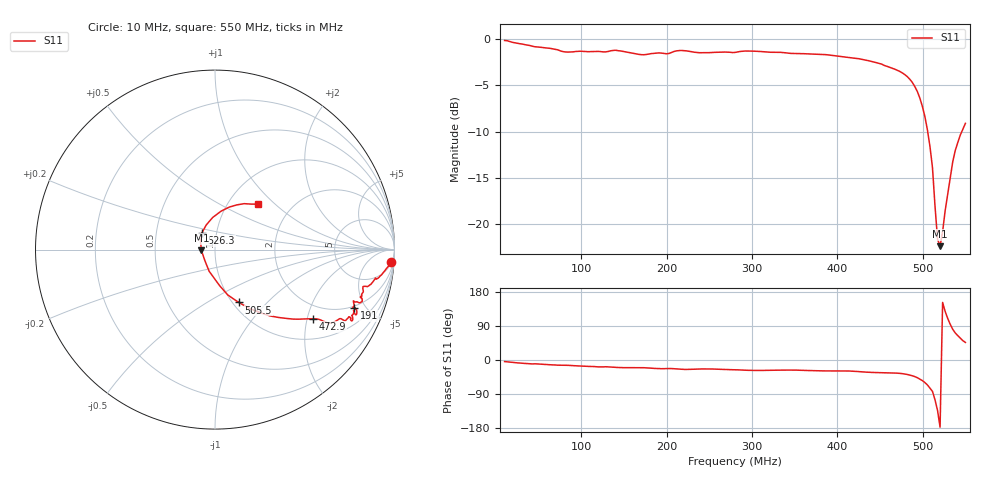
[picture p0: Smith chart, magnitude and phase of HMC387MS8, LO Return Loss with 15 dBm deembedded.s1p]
!Hittite Microwave Corporation
!12 Elizabeth Drive
!Chelmsford, MA 01824
!Tel: 978-250-3343
!Fax: 978-250-3373
!Device: HMC387MS8, 450-500 MHz, GaAs MMIC High IP3 Mixer in 8-lead plastic SMT package
!Misc: LO Return Loss with 15 dBm, Room
# MHZ S MA R 50
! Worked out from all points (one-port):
!   183 points, 10 MHz to 550 MHz, reference 50 ohm
!   lowest |S11| = -22.4 dB at 520.3 MHz (marker M1), VSWR 1.16, Z = 42.9 - j0.309 ohm
!   |S11| at or under -10 dB: 505.8 MHz to 545.8 MHz (40 MHz wide, 7.61 % of centre)
!   S11 on the Smith chart (normalised r, x): 10 MHz: 7, -26; 191 MHz: 1.87, -4.16; 472.9 MHz: 1.56, -2.18; 505.5 MHz: 1.07, -0.70; 526.3 MHz: 0.85, +0.16; 550 MHz: 1.37, +0.79
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10  0.982 -4.1
36.703  0.927 -9.6
78.242  0.855 -13.8
146.484  0.861 -20.1
173.187  0.822 -20.4
190.989  0.841 -22.8
202.857  0.836 -22.5
214.725  0.866 -24.2
250.33  0.844 -23.6
280  0.846 -25.7
303.736  0.859 -27.5
348.242  0.835 -26.6
380.879  0.827 -28.7
416.484  0.791 -29.3
440.22  0.756 -32.8
472.857  0.669 -35.2
484.725  0.607 -39.7
496.593  0.48 -50.3
505.495  0.323 -65.8
511.429  0.202 -82.8
514.396  0.125 -105.2
517.363  0.083 -133.1
520.33  0.076 -177.3
523.297  0.091 151.9
526.264  0.118 128.3
535.165  0.217 81.0
538.132  0.25 71.4
550  0.35 46.3
